[IBIS Ver]   5.0
[File name]   f28p551yaf.ibs
[File Rev]   1.0
[Date]   November 10,2025
[Source]   File originated at Texas Instruments
[Copyright]   (c) 2012, Texas Instruments Inc.
[Component]   f28p551yaf
[Manufacturer]  Texas Instruments
[Package]
| Variable   Typ   Min   Max
R_pkg  1.17E-01  2.24E-02  4.06E-01
L_pkg  7.08E-10  1.20E-10  3.05E-9
C_pkg  8.40E-14  5.54E-14  1.44E-13
[Pin]   signal_name   model_name   R_pin   L_pin   C_pin
A1   XRSn   BQ0491FS_USF   0.090037   2.425e-10   5.959e-14
A2   VSS   NC
A3   A6,B2,C6,D14,E12,E14,GPIO226 BCF3385DSHYPBFZ_LC_USF   0.049066   2.56e-10   7.464e-14
A4   A2,B6,C9,GPIO224,PGA1_INP   BCF3385DSHYPBFZ_LC   0.04777   2.142e-10   5.816e-14
A5   A15,B9,C9,PGA1_INM   BCF3385DSHYPBFZ_LC   0.037221   2.097e-10   6.861e-14
A6   A11,B10,C0,PGA2_OUT   ICF33SHYPB_LC   0.045861   1.777e-10   5.536e-14
A7   A13,B13,C13,D13,E13,VREFLO   ICF33SHYPB_LC   8.99E-02  4.94E-09   8.11E-15
B1   GPIO6   BCF3385DSHYPBFZ_LC_USF   0.063304   3.964e-10   7.084e-14
B2   GPIO48   BCF3385DSHYPBFZ_LC   0.11027   4.458e-10   7.773e-14
B3   GPIO49   BCF3385DSHYPBFZ_LC   0.1076   4.445e-10   7.695e-14
B4   A3,B3,C5,GPIO242,PGA2_INP   BCF3385DSHYPBFZ_LC_USF   0.14966   6.373e-10   8.216e-14
B5   A1,B7,D11,DACB_OUT   ICF33SHYPB_LC   0.14194   9.429e-10   8.101e-14
B6   D20,E20,VREFHI   ICF33SHYPB_LC   8.94E-02  4.90E-09   8.04E-15
B7   A8,B0,C11,PGA3_OUT   ICF33SHYPB_LC   0.022369   1.196e-10   7.332e-14
C1   GPIO5   BCF3385DSHYPBFZ_LC   0.060486   1.784e-10   5.669e-14
C2   GPIO9   BQ3320HYPBFZ_3VSBLK_5FS_LC  0.14001   9.405e-10   7.005e-14
C3   GPIO41   BCF3385DSHYPBFZ_LC   0.17862   1.333e-9   1.253e-13
C4   A14,B14,C4,PGA1_OUT   ICF33SHYPB_LC   0.12784   9.321e-10   1.127e-13
C5   A5,B12,C2,PGA2_INM   ICF33SHYPB_LC   0.17758   1.23e-9   1.253e-13
C6   A0,B15,C15,DACA_OUT   ICF33SHYPB_LC   0.14803   9.773e-10   9.682e-14
C7   VSSA   NC
D1   VDD   NC
D2   VDDA   NC
D3   GPIO40   BCF3385DSHYPBFZ_LC   0.24218   1.769e-9   9.019e-14
D4   VSS   NC
D5   A12,C1,E11,PGA3_INP   ICF33SHYPB_LC   0.12036   8.577e-10   1.442e-13
D6   A7,B30,C3,D12,E0,PGA3_INM   ICF33SHYPB_LC   0.090489   6.326e-10   1.311e-13
D7   VDDA   NC
E1   GPIO0   BCF3385DSHYPBFZ_LC   0.1021   3.176e-10   9.266e-14
E2   GPIO3   BQ3320HYPBFZ_3VSBLK_5FS_LC  0.24591   1.757e-9   8.571e-14
E3   A24,D0,E0,GPIO11   BCF3385DSHYPBFZ_LC   0.40567   3.052e-9   1.072e-13
E4   TMS   BCF3355DSHYPBFZ_TMS   0.16419   8.918e-10   1.099e-13
E5   GPIO37/TDO   BCPF335585DSHYPBFZ   0.23265   1.521e-9   7.579e-14
E6   A10,A9,B1,C20,GPIO227,GPIO230 BCF3385DSHYPBFZ_LC   0.08067   5.396e-10   8.793e-14
E7   A4,B8,C14   ICF33SHYPB_LC   0.058525   3.379e-10   8.35e-14
F1   GPIO1   BCF3385DSHYPBFZ_LC   0.0603   1.79e-10   5.679e-14
F2   GPIO4   BCF3385DSHYPBFZ_LC   0.25852   1.414e-9   8.298e-14
F3   VDDIO   NC
F4   VSS   NC
F5   GPIO32   BQ3320HYPBFZ_3VSBLK_5FS_LC  0.14572   1.001e-9   8.301e-14
F6   A17,B17,C17,CMP1_DACL,GPIO20  BCF3385DSHYPBFZ_LC   0.071958   4.27e-10   7.571e-14
F7   VSS   NC
G1   VSS   NC
G2   VDD   NC
G3   GPIO19,X1   BCPF335585DSHYPBFZ   0.056279   1.764e-10   7.562e-14
G4   GPIO18,X2   BCF3385DSHYPBFZ_LC   0.029705   1.733e-10   7.727e-14
G5   GPIO35/TDI   BCF3385DSHYPBFZ_LC   0.062414   2.235e-10   7.016e-14
G6   TCK   BCF3355DSHYPBFZ_TMS_USF  0.0464   2.377e-10   6.814e-14
G7   B25,D4,E4,GPIO24   BCF3385DSHYPBFZ_LC   0.051092   2.883e-10   6.195e-14
| End of package information
|   Component BQ0491FS_USF
[Component]   BQ0491FS_USF
[Manufacturer]   Texas Instruments
[Package]
|  variable   typ   min   max
R_pkg   0   0   0
L_pkg   0   0   0
C_pkg   0   0   0
[Pin]   signal_name   model_name   R_pin   L_pin   C_pin
VSS   VSS   GND
VDDS   VDDS   POWER
PAD   PAD   BQ0491FS_USF
[Model Selector] BQ0491FS_USF
WK_PU_ON_WITH_RX_3P3  Cell operated at 3.3(nom)
|WK_PU_ON_WITH_RX_3P3; WEAK_PULLUP_ON_WITH_RX
OPEN_DRAIN_MODE_3P3  Cell operated at 3.3(nom)
|   Component BCPF335585DSHYPBFZ
[Component]   BCPF335585DSHYPBFZ
[Manufacturer]   Texas Instruments
[Package]
|  variable   typ   min   max
R_pkg   0   0   0
L_pkg   0   0   0
C_pkg   0   0   0
[Pin]   signal_name   model_name   R_pin   L_pin   C_pin
VSS   VSS   GND
VDDS   VDDS   POWER
PAD   PAD   BCPF335585DSHYPBFZ
[Model Selector] BCPF335585DSHYPBFZ
BCPF_WK_PU_ON_3P3  Cell operated at 3.3(nom)
|BCPF_WK_PU_ON_3P3; WEAK_PULLUP_ON
BCPF_DRIVER_MODE_4MA_3P3  Cell operated at 3.3(nom)
|BCPF_DRIVER_MODE_4MA_3P3
BCPF_DRIVER_MODE_2MA_3P3  Cell operated at 3.3(nom)
|BCPF_DRIVER_MODE_2MA_3P3
BCPF_WK_PD_ON_3P3  Cell operated at 3.3(nom)
|   Component ICF33SHYPB_LC
[Component]   ICF33SHYPB_LC
[Manufacturer]   Texas Instruments
[Package]
|  variable   typ   min   max
R_pkg   0   0   0
L_pkg   0   0   0
C_pkg   0   0   0
[Pin]   signal_name   model_name   R_pin   L_pin   C_pin
VSS   VSS   GND
VDDS   VDDS   POWER
PAD   PAD   ICF33SHYPB_LC
[Model Selector] ICF33SHYPB_LC
ICF_RECEIVER_MODE_3P3  Cell operated at 3.3(nom)
|ICF_RECEIVER_MODE_3P3; RECEIVER_MODE
ICF_WK_PU_ON_3P3  Cell operated at 3.3(nom)
|ICF_WK_PU_ON_3P3; WEAK_PULLUP_ON
ICF_WK_PD_ON_3P3  Cell operated at 3.3(nom)
|   Component BCF3385DSHYPBFZ_LC_USF
[Component]   BCF3385DSHYPBFZ_LC_USF
[Manufacturer]   Texas Instruments
[Package]
|  variable   typ   min   max
R_pkg   0   0   0
L_pkg   0   0   0
C_pkg   0   0   0
[Pin]   signal_name   model_name   R_pin   L_pin   C_pin
VSS   VSS   GND
VDDS   VDDS   POWER
PAD   PAD   BCF3385DSHYPBFZ_LC_USF
[Model Selector] BCF3385DSHYPBFZ_LC_USF
BCF_WK_PU_ON_3P3  Cell operated at 3.3(nom)
|BCF_WK_PU_ON_3P3; WEAK_PULLUP_ON
BCF_WK_PD_ON_3P3  Cell operated at 3.3(nom)
|BCF_WK_PD_ON_3P3; WEAK_PULLDOWN_ON
BCF_DRIVER_MODE_3P3  Cell operated at 3.3(nom)
|BCF_DRIVER_MODE_3P3
BCF_RECEIVER_MODE_3P3  Cell operated at 3.3(nom)
|   Component BCF3355DSHYPBFZ_TMS_USF
[Component]   BCF3355DSHYPBFZ_TMS_USF
[Manufacturer]   Texas Instruments
[Package]
|  variable   typ   min   max
R_pkg   0   0   0
L_pkg   0   0   0
C_pkg   0   0   0
[Pin]   signal_name   model_name   R_pin   L_pin   C_pin
VSS   VSS   GND
VDDS   VDDS   POWER
PAD   PAD   BCF3355DSHYPBFZ_TMS_USF
[Model Selector] BCF3355DSHYPBFZ_TMS_USF
TMS_WK_PU_ON_3P3  Cell operated at 3.3(nom)
|TMS_WK_PU_ON_3P3; WEAK_PULLUP_ON
TMS_DRIVER_3P3  Cell operated at 3.3(nom)
|TMS_DRIVER_3P3
TMS_WK_PD_ON_3P3  Cell operated at 3.3(nom)
|   Component BCF3385DSHYPBFZ_LC
[Component]   BCF3385DSHYPBFZ_LC
[Manufacturer]   Texas Instruments
[Package]
|  variable   typ   min   max
R_pkg   0   0   0
L_pkg   0   0   0
C_pkg   0   0   0
[Pin]   signal_name   model_name   R_pin   L_pin   C_pin
VSS   VSS   GND
VDDS   VDDS   POWER
PAD   PAD   BCF3385DSHYPBFZ_LC
[Model Selector] BCF3385DSHYPBFZ_LC
BCF_WK_PU_ON_3P3  Cell operated at 3.3(nom)
|BCF_WK_PU_ON_3P3; WEAK_PULLUP_ON
BCF_WK_PD_ON_3P3  Cell operated at 3.3(nom)
|BCF_WK_PD_ON_3P3; WEAK_PULLDOWN_ON
BCF_DRIVER_MODE_3P3  Cell operated at 3.3(nom)
|BCF_DRIVER_MODE_3P3
BCF_RECEIVER_MODE_3P3  Cell operated at 3.3(nom)
|BCF_RECEIVER_MODE_3P3; RECEIVER_MODE
|   Component IQ0440FS_VREGENZ_USF
[Component]   IQ0440FS_VREGENZ_USF
[Manufacturer]   Texas Instruments
[Package]
|  variable   typ   min   max
R_pkg   0   0   0
L_pkg   0   0   0
C_pkg   0   0   0
[Pin]   signal_name   model_name   R_pin   L_pin   C_pin
VSS   VSS   GND
VDDS   VDDS   POWER
PAD   PAD   IQ0440FS_VREGENZ_USF
[Model Selector] IQ0440FS_VREGENZ_USF
VREGENZ_WK_PD_ON_3P3  Cell operated at 3.3(nom)
|VREGENZ_WK_PD_ON_3P3; WEAK_PULLDOWN_ON
VREGENZ_WK_PD_OFF_3P3  Cell operated at 3.3(nom)
|   Component BCF3355DSHYPBFZ_TMS
[Component]   BCF3355DSHYPBFZ_TMS
[Manufacturer]   Texas Instruments
[Package]
|  variable   typ   min   max
R_pkg   0   0   0
L_pkg   0   0   0
C_pkg   0   0   0
[Pin]   signal_name   model_name   R_pin   L_pin   C_pin
VSS   VSS   GND
VDDS   VDDS   POWER
PAD   PAD   BCF3355DSHYPBFZ_TMS
[Model Selector] BCF3355DSHYPBFZ_TMS
TMS_WK_PU_ON_3P3  Cell operated at 3.3(nom)
|TMS_WK_PU_ON_3P3; WEAK_PULLUP_ON
TMS_DRIVER_3P3  Cell operated at 3.3(nom)
|TMS_DRIVER_3P3
TMS_WK_PD_ON_3P3  Cell operated at 3.3(nom)
|TMS_WK_PD_ON_3P3; WEAK_PULLDOWN_ON
|   Component BQ3320HYPBFZ_3VSBLK_5FS_LC
[Component] BQ3320HYPBFZ_3VSBLK_5FS_LC
[Manufacturer] Texas Instruments
[Package]
| variable   typ   min   max
R_pkg   0.0   0.0   0.0
L_pkg   0.0H   0.0H   0.0H
C_pkg   0.0F   0.0F   0.0F
[Pin]  signal_name   model_name   R_pin   L_pin   C_pin
PAD   PAD   BQ3320HYPBFZ_3VSBLK_5FS_LC
VDDS   VDDS   Power
VSS   VSS   Gnd
A   A   NC
GZ   GZ   NC
[Model Selector] BQ3320HYPBFZ_3VSBLK_5FS_LC
BQ3320HYPBFZ_3VSBLK_5FS_LC_M0_D0 I/O model with Mode = 0 and Drive = 0
BQ3320HYPBFZ_3VSBLK_5FS_LC_M0_D1 I/O model with Mode = 0 and Drive = 1
BQ3320HYPBFZ_3VSBLK_5FS_LC_M1_D0 I/O model with Mode = 1 and Drive = 0
BQ3320HYPBFZ_3VSBLK_5FS_LC_M1_D1 I/O model with Mode = 1 and Drive = 1
BQ3320HYPBFZ_3VSBLK_5FS_LC_PDON I/O model with Pulldown on PI=0 PSEL=0
BQ3320HYPBFZ_3VSBLK_5FS_LC_PUON I/O model with Pullup on PI=0 PSEL=0
| Models and submodels in the file (24): WK_PU_ON_WITH_RX_3P3 (Input), OPEN_DRAIN_MODE_3P3 (I/O_open_drain), BCPF_WK_PU_ON_3P3 (Input), BCPF_DRIVER_MODE_4MA_3P3 (I/O), BCPF_DRIVER_MODE_2MA_3P3 (I/O), BCPF_WK_PD_ON_3P3 (Input), ICF_RECEIVER_MODE_3P3 (Input), ICF_WK_PU_ON_3P3 (Input), ICF_WK_PD_ON_3P3 (Input), BCF_WK_PU_ON_3P3 (Input), BCF_WK_PD_ON_3P3 (Input), BCF_DRIVER_MODE_3P3 (I/O), BCF_RECEIVER_MODE_3P3 (Input), TMS_WK_PU_ON_3P3 (Input), TMS_DRIVER_3P3 (I/O), TMS_WK_PD_ON_3P3 (Input), VREGENZ_WK_PD_ON_3P3 (Input), VREGENZ_WK_PD_OFF_3P3 (Input), BQ3320HYPBFZ_3VSBLK_5FS_LC_M0_D0 (I/O), BQ3320HYPBFZ_3VSBLK_5FS_LC_M0_D1 (I/O), BQ3320HYPBFZ_3VSBLK_5FS_LC_M1_D0 (I/O), BQ3320HYPBFZ_3VSBLK_5FS_LC_M1_D1 (I/O), BQ3320HYPBFZ_3VSBLK_5FS_LC_PDON (Input), BQ3320HYPBFZ_3VSBLK_5FS_LC_PUON (Input)
